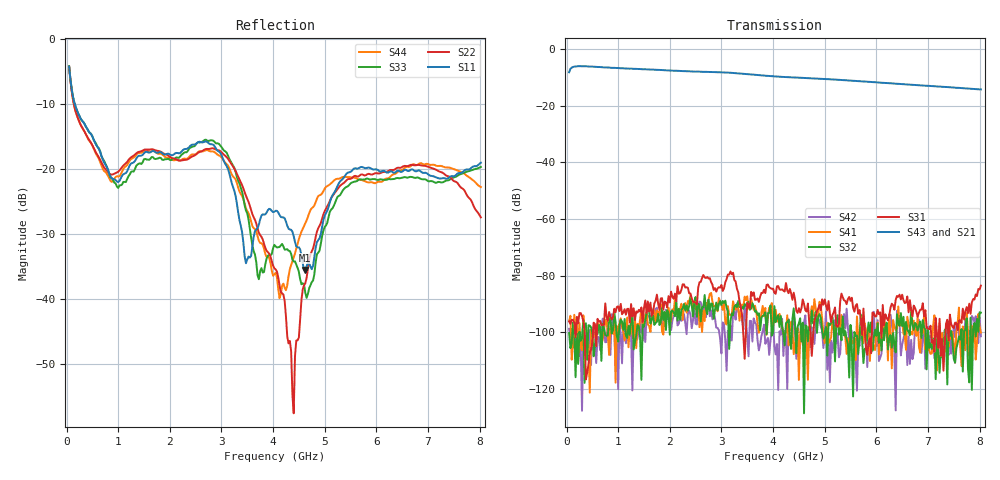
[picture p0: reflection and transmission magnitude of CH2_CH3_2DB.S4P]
!Agilent Technologies,E5071C,MY46316741,A.11.02
!Date: Thu May 28 14:39:33 2026
!Data & Calibration Information:
!1:CH2 INPUT 2:CH2 OUTPUT 3:CH3 INPUT 4:CH3 OUTPUT
!Freq	S11:SOLT4(ON)	S12:SOLT4(ON)	S13:SOLT4(ON)	S14:SOLT4(ON)
!	S21:SOLT4(ON)	S22:SOLT4(ON)	S23:SOLT4(ON)	S24:SOLT4(ON)
!	S31:SOLT4(ON)	S32:SOLT4(ON)	S33:SOLT4(ON)	S34:SOLT4(ON)
!	S41:SOLT4(ON)	S42:SOLT4(ON)	S43:SOLT4(ON)	S44:SOLT4(ON)
!PortZ  Port1:50+j0  Port2:50+j0  Port3:50+j0  Port4:50+j0
!Above PortZ is port z conversion or system Z0 setting when saving the data.
!When reading, reference impedance value at option line is always used.
# Hz S dB R 50
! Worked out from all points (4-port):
!   320 points, 50 MHz to 8.025 GHz, reference 50 ohm
!   strongest paths, dB at 50 MHz, 2.05 GHz, 4.05 GHz, 6.05 GHz, 8.025 GHz:
!     S43: -8.2, -7.6, -9.7, -11.9, -14.3
!     S21: -8.3, -7.8, -10.0, -12.1, -14.5
!     S31: -96.1, -87.4, -86.4, -93.5, -83.5
!     S32: -100.2, -92.3, -96.4, -103.7, -93.0
!     S41: -96.0, -91.8, -92.0, -107.8, -100.0
!     S42: -98.7, -95.8, -107.7, -110.1, -101.4
!   lowest |S11| = -35.5 dB at 4.625 GHz (marker M1), VSWR 1.03, Z = 51.4 + j0.956 ohm
!   |S11| at or under -10 dB: 158.5 MHz to end of sweep
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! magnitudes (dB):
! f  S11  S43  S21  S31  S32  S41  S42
! 50 MHz  -4.3  -8.2  -8.3  -96.1  -100.2  -96.0  -98.7
! 1 GHz  -22.0  -6.7  -6.9  -90.8  -103.2  -99.3  -120.0
! 3.15 GHz  -20.6  -8.4  -8.6  -79.6  -105.8  -93.8  -104.6
! 4.4 GHz  -30.3  -10.1  -10.3  -86.0  -91.5  -107.6  -93.3
! 4.625 GHz  -35.5  -10.3  -10.5  -92.1  -97.5  -98.9  -94.0
! 5.575 GHz  -19.9  -11.3  -11.5  -92.7  -99.8  -102.1  -101.9
! 8.025 GHz  -19.0  -14.3  -14.5  -83.5  -93.0  -100.0  -101.4
